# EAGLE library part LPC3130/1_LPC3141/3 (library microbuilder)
LPC3130/LPC3131 - 180MHz ARM926EJ-S CPU with 96KB (LPC3130) or 192KB (LPC3131) SRAM LPC3141 - 270MHz ARM926EJ-S CPU with 192KB SRAM LPC3143 - 270MHz ARM926EJ-S CPU with 192KB SRAM and AES decryption engine/128-bit unique ID (LPC3143 only)
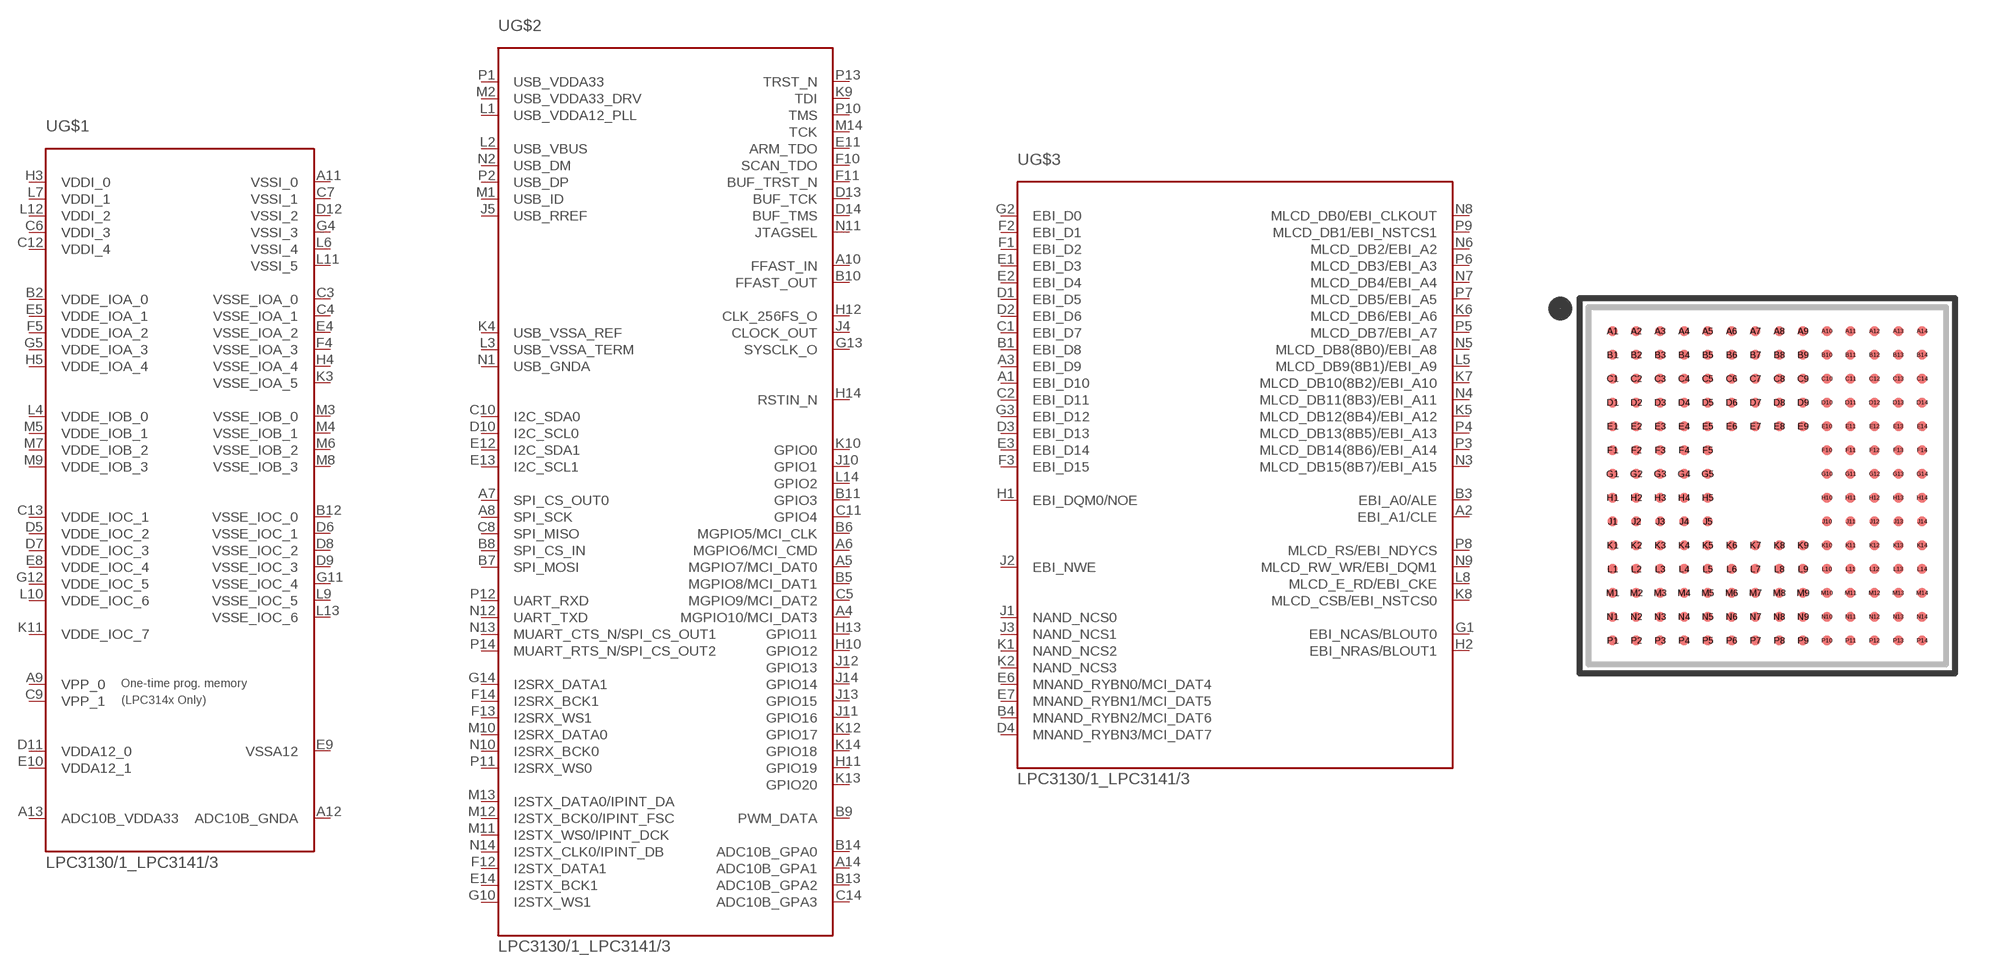
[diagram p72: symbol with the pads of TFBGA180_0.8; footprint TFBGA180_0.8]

Designator prefix U; gates G$1=LPC313X/314X_0 G$2=LPC313X/314X_1 G$3=LPC313X/314X_2

## LPC3130/1_LPC3141/3  [TFBGA180_0.8]
A1  G$3:EBI_D10
A2  G$3:EBI_A1/CLE
A3  G$3:EBI_D9
A4  G$2:MGPIO10/MCI_DAT3
A5  G$2:MGPIO7/MCI_DAT0
A6  G$2:MGPIO6/MCI_CMD
A7  G$2:SPI_CS_OUT0
A8  G$2:SPI_SCK
A9  G$1:VPP_0  pwr
A10  G$2:FFAST_IN
A11  G$1:VSSI_0  pwr
A12  G$1:ADC10B_GNDA  pwr
A13  G$1:ADC10B_VDDA33  pwr
A14  G$2:ADC10B_GPA1
B1  G$3:EBI_D8
B2  G$1:VDDE_IOA_0  pwr
B3  G$3:EBI_A0/ALE
B4  G$3:MNAND_RYBN2/MCI_DAT6
B5  G$2:MGPIO8/MCI_DAT1
B6  G$2:MGPIO5/MCI_CLK
B7  G$2:SPI_MOSI
B8  G$2:SPI_CS_IN
B9  G$2:PWM_DATA
B10  G$2:FFAST_OUT
B11  G$2:GPIO3
B12  G$1:VSSE_IOC_0  pwr
B13  G$2:ADC10B_GPA2
B14  G$2:ADC10B_GPA0
C1  G$3:EBI_D7
C2  G$3:EBI_D11
C3  G$1:VSSE_IOA_0  pwr
C4  G$1:VSSE_IOA_1  pwr
C5  G$2:MGPIO9/MCI_DAT2
C6  G$1:VDDI_3  pwr
C7  G$1:VSSI_1  pwr
C8  G$2:SPI_MISO
C9  G$1:VPP_1  pwr
C10  G$2:I2C_SDA0
C11  G$2:GPIO4
C12  G$1:VDDI_4  pwr
C13  G$1:VDDE_IOC_1  pwr
C14  G$2:ADC10B_GPA3
D1  G$3:EBI_D5
D2  G$3:EBI_D6
D3  G$3:EBI_D13
D4  G$3:MNAND_RYBN3/MCI_DAT7
D5  G$1:VDDE_IOC_2  pwr
D6  G$1:VSSE_IOC_1  pwr
D7  G$1:VDDE_IOC_3  pwr
D8  G$1:VSSE_IOC_2  pwr
D9  G$1:VSSE_IOC_3  pwr
D10  G$2:I2C_SCL0
D11  G$1:VDDA12_0  pwr
D12  G$1:VSSI_2  pwr
D13  G$2:BUF_TCK
D14  G$2:BUF_TMS
E1  G$3:EBI_D3
E2  G$3:EBI_D4
E3  G$3:EBI_D14
E4  G$1:VSSE_IOA_2  pwr
E5  G$1:VDDE_IOA_1  pwr
E6  G$3:MNAND_RYBN0/MCI_DAT4
E7  G$3:MNAND_RYBN1/MCI_DAT5
E8  G$1:VDDE_IOC_4  pwr
E9  G$1:VSSA12  pwr
E10  G$1:VDDA12_1  pwr
E11  G$2:ARM_TDO
E12  G$2:I2C_SDA1
E13  G$2:I2C_SCL1
E14  G$2:I2STX_BCK1
F1  G$3:EBI_D2
F2  G$3:EBI_D1
F3  G$3:EBI_D15
F4  G$1:VSSE_IOA_3  pwr
F5  G$1:VDDE_IOA_2  pwr
F10  G$2:SCAN_TDO
F11  G$2:BUF_TRST_N
F12  G$2:I2STX_DATA1
F13  G$2:I2SRX_WS1
F14  G$2:I2SRX_BCK1
G1  G$3:EBI_NCAS/BLOUT0
G2  G$3:EBI_D0
G3  G$3:EBI_D12
G4  G$1:VSSI_3  pwr
G5  G$1:VDDE_IOA_3  pwr
G10  G$2:I2STX_WS1
G11  G$1:VSSE_IOC_4  pwr
G12  G$1:VDDE_IOC_5  pwr
G13  G$2:SYSCLK_O
G14  G$2:I2SRX_DATA1
H1  G$3:EBI_DQM0/NOE
H2  G$3:EBI_NRAS/BLOUT1
H3  G$1:VDDI_0  pwr
H4  G$1:VSSE_IOA_4  pwr
H5  G$1:VDDE_IOA_4  pwr
H10  G$2:GPIO12
H11  G$2:GPIO19
H12  G$2:CLK_256FS_O
H13  G$2:GPIO11
H14  G$2:RSTIN_N
J1  G$3:NAND_NCS0
J2  G$3:EBI_NWE
J3  G$3:NAND_NCS1
J4  G$2:CLOCK_OUT
J5  G$2:USB_RREF
J10  G$2:GPIO1
J11  G$2:GPIO16
J12  G$2:GPIO13
J13  G$2:GPIO15
J14  G$2:GPIO14
K1  G$3:NAND_NCS2
K2  G$3:NAND_NCS3
K3  G$1:VSSE_IOA_5  pwr
K4  G$2:USB_VSSA_REF
K5  G$3:MLCD_DB12(8B4)/EBI_A12
K6  G$3:MLCD_DB6/EBI_A6
K7  G$3:MLCD_DB10(8B2)/EBI_A10
K8  G$3:MLCD_CSB/EBI_NSTCS0
K9  G$2:TDI
K10  G$2:GPIO0
K11  G$1:VDDE_IOC_7  pwr
K12  G$2:GPIO17
K13  G$2:GPIO20
K14  G$2:GPIO18
L1  G$2:USB_VDDA12_PLL
L2  G$2:USB_VBUS
L3  G$2:USB_VSSA_TERM
L4  G$1:VDDE_IOB_0  pwr
L5  G$3:MLCD_DB9(8B1)/EBI_A9
L6  G$1:VSSI_4  pwr
L7  G$1:VDDI_1  pwr
L8  G$3:MLCD_E_RD/EBI_CKE
L9  G$1:VSSE_IOC_5  pwr
L10  G$1:VDDE_IOC_6  pwr
L11  G$1:VSSI_5  pwr
L12  G$1:VDDI_2  pwr
L13  G$1:VSSE_IOC_6  pwr
L14  G$2:GPIO2
M1  G$2:USB_ID
M2  G$2:USB_VDDA33_DRV
M3  G$1:VSSE_IOB_0  pwr
M4  G$1:VSSE_IOB_1  pwr
M5  G$1:VDDE_IOB_1  pwr
M6  G$1:VSSE_IOB_2  pwr
M7  G$1:VDDE_IOB_2  pwr
M8  G$1:VSSE_IOB_3  pwr
M9  G$1:VDDE_IOB_3  pwr
M10  G$2:I2SRX_DATA0
M11  G$2:I2STX_WS0/IPINT_DCK
M12  G$2:I2STX_BCK0/IPINT_FSC
M13  G$2:I2STX_DATA0/IPINT_DA
M14  G$2:TCK
N1  G$2:USB_GNDA
N2  G$2:USB_DM
N3  G$3:MLCD_DB15(8B7)/EBI_A15
N4  G$3:MLCD_DB11(8B3)/EBI_A11
N5  G$3:MLCD_DB8(8B0)/EBI_A8
N6  G$3:MLCD_DB2/EBI_A2
N7  G$3:MLCD_DB4/EBI_A4
N8  G$3:MLCD_DB0/EBI_CLKOUT
N9  G$3:MLCD_RW_WR/EBI_DQM1
N10  G$2:I2SRX_BCK0
N11  G$2:JTAGSEL
N12  G$2:UART_TXD
N13  G$2:MUART_CTS_N/SPI_CS_OUT1
N14  G$2:I2STX_CLK0/IPINT_DB
P1  G$2:USB_VDDA33
P2  G$2:USB_DP
P3  G$3:MLCD_DB14(8B6)/EBI_A14
P4  G$3:MLCD_DB13(8B5)/EBI_A13
P5  G$3:MLCD_DB7/EBI_A7
P6  G$3:MLCD_DB3/EBI_A3
P7  G$3:MLCD_DB5/EBI_A5
P8  G$3:MLCD_RS/EBI_NDYCS
P9  G$3:MLCD_DB1/EBI_NSTCS1
P10  G$2:TMS
P11  G$2:I2SRX_WS0
P12  G$2:UART_RXD
P13  G$2:TRST_N
P14  G$2:MUART_RTS_N/SPI_CS_OUT2

## Footprint TFBGA180_0.8 (pad centres in mm)
TFBGA180 (12.0x12.0mm, 0.8mm pitch, 0.45mm balls) Source: http://ics.nxp.com/products/lpc3000/datasheet/lpc3130.lpc3131.pdf Pad size is 0.34mm copper and ~0.5mm total with the solder mask (which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
smd 0.34 x 0.34: A1 -5.2,5.2; A2 -4.4,5.2; A3 -3.6,5.2; A4 -2.8,5.2; A5 -2,5.2; A6 -1.2,5.2; A7 -0.4,5.2; A8 0.4,5.2; A9 1.2,5.2; A10 2,5.2; A11 2.8,5.2; A12 3.6,5.2; A13 4.4,5.2; A14 5.2,5.2; B1 -5.2,4.4; B2 -4.4,4.4; B3 -3.6,4.4; B4 -2.8,4.4; B5 -2,4.4; B6 -1.2,4.4; B7 -0.4,4.4; B8 0.4,4.4; B9 1.2,4.4; B10 2,4.4; B11 2.8,4.4; B12 3.6,4.4; B13 4.4,4.4; B14 5.2,4.4; C1 -5.2,3.6; C2 -4.4,3.6; C3 -3.6,3.6; C4 -2.8,3.6; C5 -2,3.6; C6 -1.2,3.6; C7 -0.4,3.6; C8 0.4,3.6; C9 1.2,3.6; C10 2,3.6; C11 2.8,3.6; C12 3.6,3.6; C13 4.4,3.6; C14 5.2,3.6; D1 -5.2,2.8; D2 -4.4,2.8; D3 -3.6,2.8; D4 -2.8,2.8; D5 -2,2.8; D6 -1.2,2.8; D7 -0.4,2.8; D8 0.4,2.8; D9 1.2,2.8; D10 2,2.8; D11 2.8,2.8; D12 3.6,2.8; D13 4.4,2.8; D14 5.2,2.8; E1 -5.2,2; E2 -4.4,2; E3 -3.6,2; E4 -2.8,2; E5 -2,2; E6 -1.2,2; E7 -0.4,2; E8 0.4,2; E9 1.2,2; E10 2,2; E11 2.8,2; E12 3.6,2; E13 4.4,2; E14 5.2,2; F1 -5.2,1.2; F2 -4.4,1.2; F3 -3.6,1.2; F4 -2.8,1.2; F5 -2,1.2; F10 2,1.2; F11 2.8,1.2; F12 3.6,1.2; F13 4.4,1.2; F14 5.2,1.2; G1 -5.2,0.4; G2 -4.4,0.4; G3 -3.6,0.4; G4 -2.8,0.4; G5 -2,0.4; G10 2,0.4; G11 2.8,0.4; G12 3.6,0.4; G13 4.4,0.4; G14 5.2,0.4; H1 -5.2,-0.4; H2 -4.4,-0.4; H3 -3.6,-0.4; H4 -2.8,-0.4; H5 -2,-0.4; H10 2,-0.4; H11 2.8,-0.4; H12 3.6,-0.4; H13 4.4,-0.4; H14 5.2,-0.4; J1 -5.2,-1.2; J2 -4.4,-1.2; J3 -3.6,-1.2; J4 -2.8,-1.2; J5 -2,-1.2; J10 2,-1.2; J11 2.8,-1.2; J12 3.6,-1.2; J13 4.4,-1.2; J14 5.2,-1.2; K1 -5.2,-2; K2 -4.4,-2; K3 -3.6,-2; K4 -2.8,-2; K5 -2,-2; K6 -1.2,-2; K7 -0.4,-2; K8 0.4,-2; K9 1.2,-2; K10 2,-2; K11 2.8,-2; K12 3.6,-2; K13 4.4,-2; K14 5.2,-2; L1 -5.2,-2.8; L2 -4.4,-2.8; L3 -3.6,-2.8; L4 -2.8,-2.8; L5 -2,-2.8; L6 -1.2,-2.8; L7 -0.4,-2.8; L8 0.4,-2.8; L9 1.2,-2.8; L10 2,-2.8; L11 2.8,-2.8; L12 3.6,-2.8; L13 4.4,-2.8; L14 5.2,-2.8; M1 -5.2,-3.6; M2 -4.4,-3.6; M3 -3.6,-3.6; M4 -2.8,-3.6; M5 -2,-3.6; M6 -1.2,-3.6; M7 -0.4,-3.6; M8 0.4,-3.6; M9 1.2,-3.6; M10 2,-3.6; M11 2.8,-3.6; M12 3.6,-3.6; M13 4.4,-3.6; M14 5.2,-3.6; N1 -5.2,-4.4; N2 -4.4,-4.4; N3 -3.6,-4.4; N4 -2.8,-4.4; N5 -2,-4.4; N6 -1.2,-4.4; N7 -0.4,-4.4; N8 0.4,-4.4; N9 1.2,-4.4; N10 2,-4.4; N11 2.8,-4.4; N12 3.6,-4.4; N13 4.4,-4.4; N14 5.2,-4.4; P1 -5.2,-5.2; P2 -4.4,-5.2; P3 -3.6,-5.2; P4 -2.8,-5.2; P5 -2,-5.2; P6 -1.2,-5.2; P7 -0.4,-5.2; P8 0.4,-5.2; P9 1.2,-5.2; P10 2,-5.2; P11 2.8,-5.2; P12 3.6,-5.2; P13 4.4,-5.2; P14 5.2,-5.2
